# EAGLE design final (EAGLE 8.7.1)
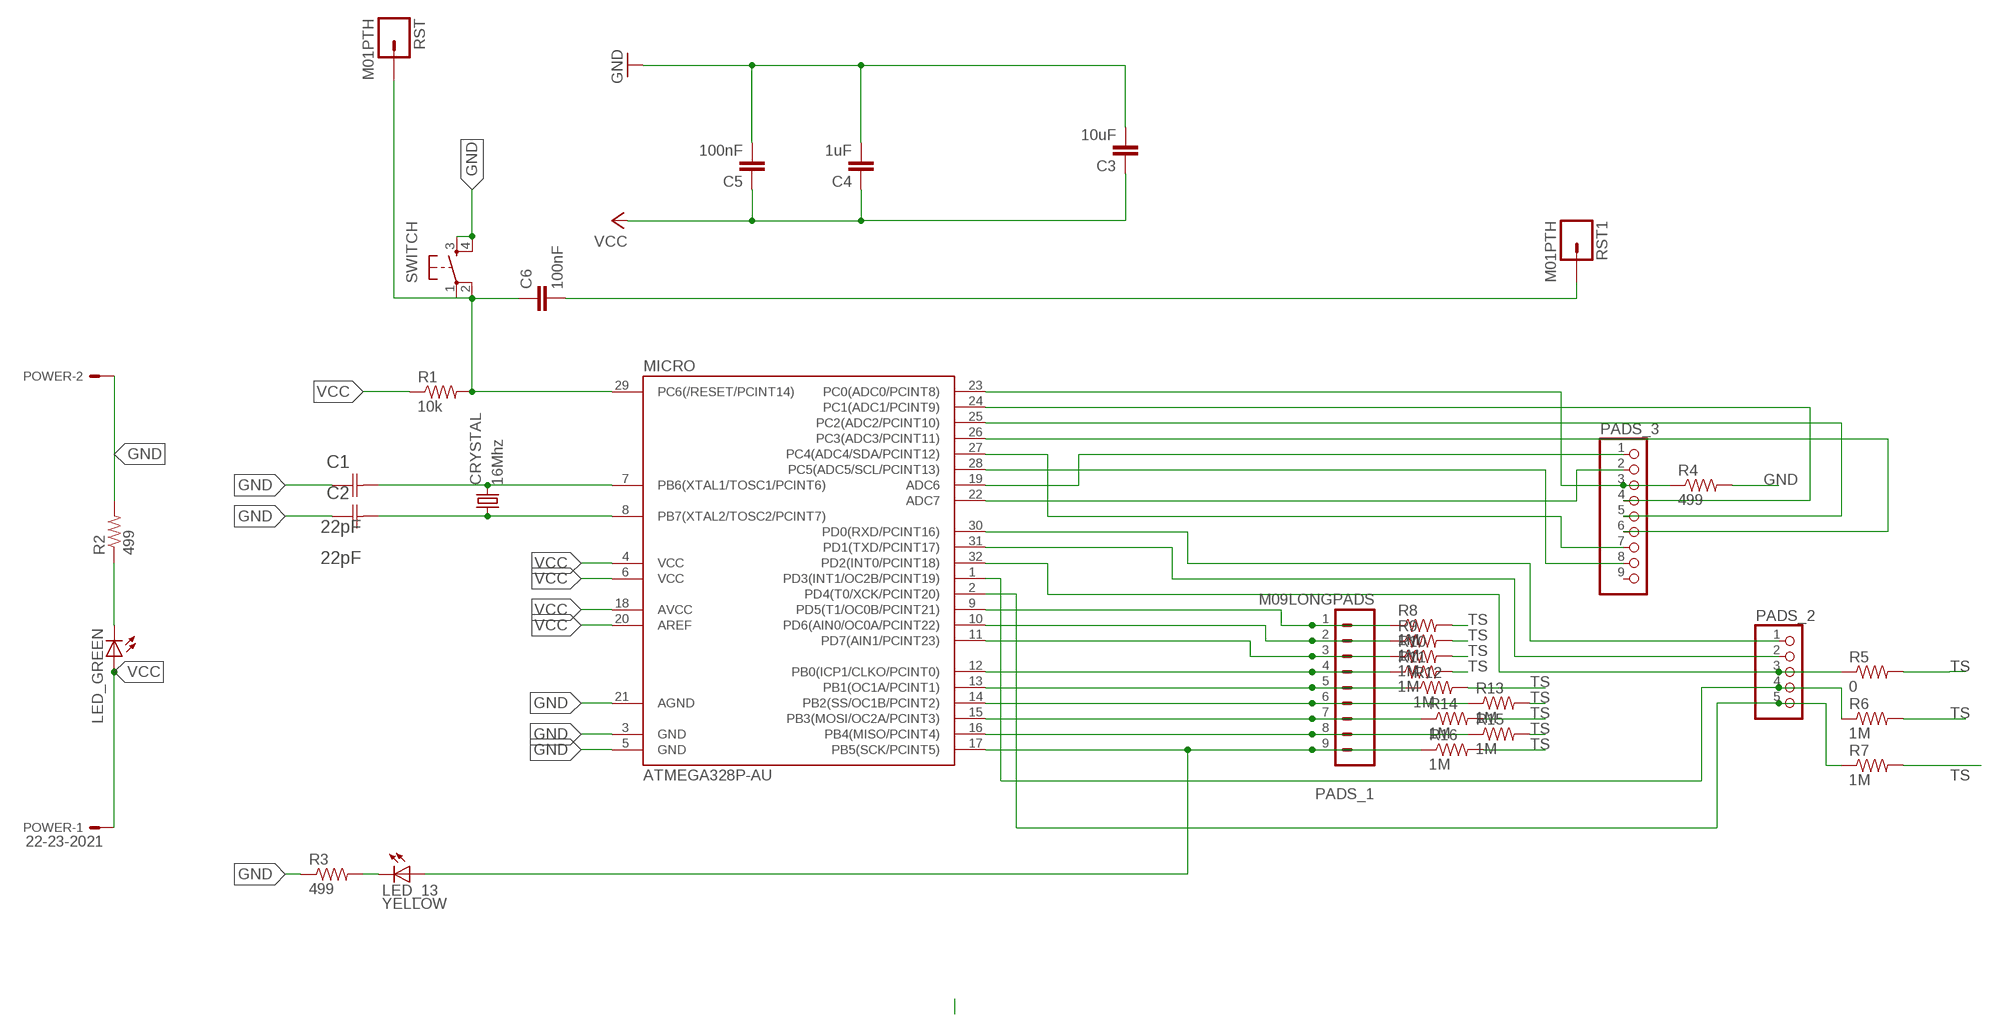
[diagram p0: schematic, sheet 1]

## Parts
C1  22pF  0612ZC225MAT2A  [CAPC3216X178N]
C2  22pF  0612ZC225MAT2A  [CAPC3216X178N]
C3  10uF  CAP1206  [1206]
C4  1uF  CAP1206  [1206]
C5  100nF  CAP1206  [1206]
C6  100nF  CAP1206  [1206]
CRYSTAL  16Mhz  CSM-7X-DU  [CSM-7X-DU]
LED_13  YELLOW  LED1206  [1206]
LED_GREEN  LED1206  [1206]
MICRO  ATMEGA328P-AU  ATMEGA48/88/168-AU  [TQFP32-08]
PADS_1  M09LONGPADS  [1X09_LONGPADS]
PADS_2  PINHD-1X5  [1X05]
PADS_3  PINHD-1X9  [1X09]
POWER  22-23-2021  [22-23-2021]
R1  10k  RESISTOR1206  [1206]
R2  499  RESISTOR1206  [1206]
R3  499  RESISTOR1206  [1206]
R4  499  RES-US1206FAB  [R1206FAB]
R5  0  RES-US1206FAB  [R1206FAB]
R6  1M  RES-US1206FAB  [R1206FAB]
R7  1M  RES-US1206FAB  [R1206FAB]
R8  1M  RES-US1206FAB  [R1206FAB]
R9  1M  RES-US1206FAB  [R1206FAB]
R10  1M  RES-US1206FAB  [R1206FAB]
R11  1M  RES-US1206FAB  [R1206FAB]
R12  1M  RES-US1206FAB  [R1206FAB]
R13  1M  RES-US1206FAB  [R1206FAB]
R14  1M  RES-US1206FAB  [R1206FAB]
R15  1M  RES-US1206FAB  [R1206FAB]
R16  1M  RES-US1206FAB  [R1206FAB]
RST  M01PTH  [1X01]
RST1  M01PTH  [1X01]
SWITCH  6MM_SWITCH6MM_SWITCH  [6MM_SWITCH]

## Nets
GND: C1.1(C1) C2.1(C1) C3.2 C4.2 C5.2 MICRO.3(GND) MICRO.5(GND) MICRO.21(AGND) POWER.2 R2.2 R3.1 R4.2 SWITCH.3(S) SWITCH.4(S1)
N$1: MICRO.9(PD5(T1/OC0B/PCINT21)) PADS_1.1 R8.1
N$2: C1.2(C2) CRYSTAL.2 MICRO.7(PB6(XTAL1/TOSC1/PCINT6))
N$4: MICRO.10(PD6(AIN0/OC0A/PCINT22)) PADS_1.2 R9.1
N$5: MICRO.11(PD7(AIN1/PCINT23)) PADS_1.3 R10.1
N$6: MICRO.12(PB0(ICP1/CLKO/PCINT0)) PADS_1.4 R11.1
N$7: MICRO.16(PB4(MISO/PCINT4)) PADS_1.8 R15.1
N$8: MICRO.15(PB3(MOSI/OC2A/PCINT3)) PADS_1.7 R14.1
N$9: C2.2(C2) CRYSTAL.1 MICRO.8(PB7(XTAL2/TOSC2/PCINT7))
N$10: MICRO.14(PB2(SS/OC1B/PCINT2)) PADS_1.6 R13.1
N$11: MICRO.13(PB1(OC1A/PCINT1)) PADS_1.5 R12.1
N$12: LED_13.1(A) MICRO.17(PB5(SCK/PCINT5)) PADS_1.9 R16.1
N$13: MICRO.19(ADC6) PADS_3.1
N$14: MICRO.22(ADC7) PADS_3.2
N$15: C6.2 RST1.1
N$16: MICRO.24(PC1(ADC1/PCINT9)) PADS_3.4
N$17: MICRO.25(PC2(ADC2/PCINT10)) PADS_3.5
N$18: MICRO.26(PC3(ADC3/PCINT11)) PADS_3.6
N$19: MICRO.27(PC4(ADC4/SDA/PCINT12)) PADS_3.7
N$20: MICRO.30(PD0(RXD/PCINT16)) PADS_2.1
N$21: MICRO.31(PD1(TXD/PCINT17)) PADS_2.2
N$25: MICRO.28(PC5(ADC5/SCL/PCINT13)) PADS_3.8
N$26: LED_GREEN.2(C) R2.1
N$27: LED_13.2(C) R3.2
N$28: C6.1 MICRO.29(PC6(/RESET/PCINT14)) R1.2 RST.1 SWITCH.1(P) SWITCH.2(P1)
N$29: MICRO.23(PC0(ADC0/PCINT8)) PADS_3.3 R4.1
N$30: MICRO.32(PD2(INT0/PCINT18)) PADS_2.3 R5.1
N$31: MICRO.1(PD3(INT1/OC2B/PCINT19)) PADS_2.4 R6.1
N$32: MICRO.2(PD4(T0/XCK/PCINT20)) PADS_2.5 R7.1
TS: R5.2 R6.2 R7.2 R8.2 R9.2 R10.2 R11.2 R12.2 R13.2 R14.2 R15.2 R16.2
VCC: C3.1 C4.1 C5.1 LED_GREEN.1(A) MICRO.4(VCC) MICRO.6(VCC) MICRO.18(AVCC) MICRO.20(AREF) POWER.1 R1.1
Unconnected: PADS_3.9

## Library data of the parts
C1 C2 = AVX_By_element14_Batch_1:0612ZC225MAT2A: Capacitor 1206; MPN: 0612ZC225MAT2A; OC_FARNELL: -; OC_NEWARK: 12N3209; SUPPLIER: AVX; TOLERANCE: ±20%; VALUE: 2.2µF; VOLTAGERATING: 10V
C3-C6 = 01_SparkFun:CAP: Capacitor
CRYSTAL = 01_FAB_Hello:CSM-7X-DU: SMD CRYSTAL; OC_FARNELL: unknown; OC_NEWARK: unknown
LED_13 LED_GREEN = 01_FAB_Hello:LED
MICRO = atmega8:ATMEGA48/88/168
PADS_1 = 01_SparkFun:M09: Header 9 Standard 9-pin 0.1" header. Use with straight break away headers (SKU : PRT-00116), right angle break away headers (PRT-00553), swiss pins (PRT-00743), machine pins (PRT-00117), and female headers (PRT-00115).
PADS_2 = pinhead:PINHD-1X5: PIN HEADER
PADS_3 = pinhead:PINHD-1X9: PIN HEADER
POWER = con-molex:22-23-2021: .100" (2.54mm) Center Header - 2 Pin; MF: MOLEX; MPN: 22-23-2021; OC_FARNELL: 1462926; OC_NEWARK: 25C3832
R1-R3 = 01_SparkFun:RESISTOR: Resistor
R4-R16 = 00fab:RES-US: Resistor (US Symbol)
RST RST1 = 01_SparkFun:M01: Header 1
SWITCH = 01_FAB_Hello:6MM_SWITCH: OMRON SWITCH

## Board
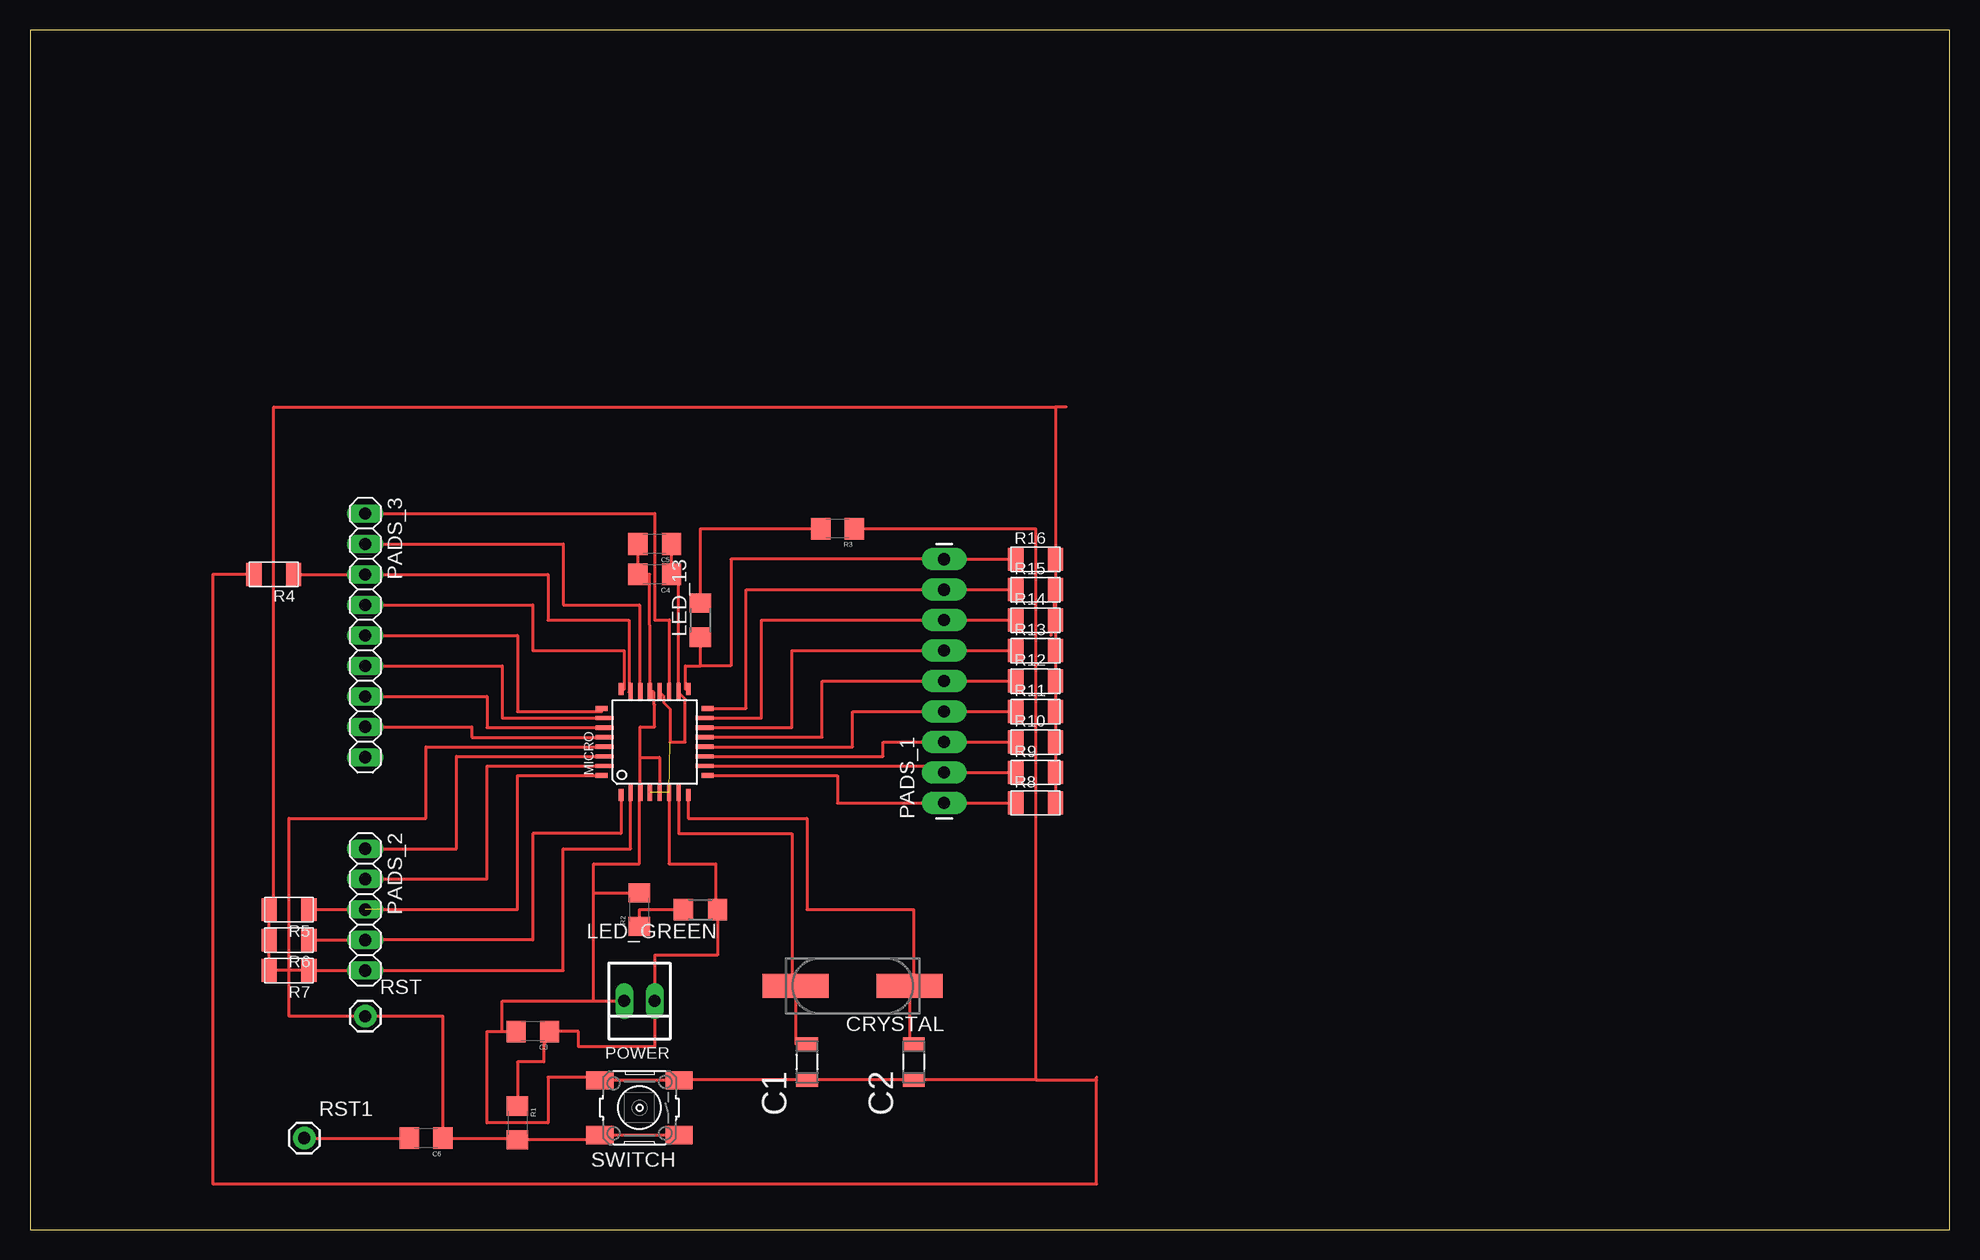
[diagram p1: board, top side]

Size 160 x 100 mm. Coordinates in mm from the lower left corner, seen from the top.
Outline: 0,0 160,0 160,100 0,100 0,0
Copper layers (1*16): Top 0.035mm / dielectric 1.5mm / Bottom 0.035mm
Design rules "default": minimum track width 6mil, minimum drill 0.35mm, track to track 6mil, track to pad 6mil, pad to pad 6mil, via to via 6mil, smd to smd 6mil, copper to edge 40mil, drill to drill 6mil, minimum pad ring 10mil, minimum via ring 8mil, stop-mask expansion 4mil, vias tented up to drill 0mil, thermal gap 10mil

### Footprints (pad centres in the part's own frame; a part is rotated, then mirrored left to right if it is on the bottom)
CAPC3216X178N = smd 1.118 x 1.803: 1 -1.499,0; 2 1.499,0
1206 = smd 1.6 x 1.8: 1 -1.4,0; 2 1.4,0
CSM-7X-DU = smd 5.5 x 2: 1 -4.75,0; 2 4.75,0
1206' = smd 1.6 x 1.803: 1 -1.422,0; 2 1.422,0
TQFP32-08 = smd 1.016 x 0.406: 1 -4.42,2.8; 8 -4.42,-2.8; 17 4.42,-2.8; 24 4.42,2.8 | smd 1.524 x 0.356: 2 -4.166,2; 3 -4.166,1.2; 4 -4.166,0.4; 5 -4.166,-0.4; 6 -4.166,-1.2; 7 -4.166,-2; 18 4.166,-2; 19 4.166,-1.2; 20 4.166,-0.4; 21 4.166,0.4; 22 4.166,1.2; 23 4.166,2 | smd 0.406 x 1.016: 9 -2.8,-4.42; 16 2.8,-4.42; 25 2.8,4.42; 32 -2.8,4.42 | smd 0.356 x 1.524: 10 -2,-4.166; 11 -1.2,-4.166; 12 -0.4,-4.166; 13 0.4,-4.166; 14 1.2,-4.166; 15 2,-4.166; 26 2,4.166; 27 1.2,4.166; 28 0.4,4.166; 29 -0.4,4.166; 30 -1.2,4.166; 31 -2,4.166
1X09_LONGPADS = drill 1.016 pad 1.88 long: 1 0,0; 2 2.54,0; 3 5.08,0; 4 7.62,0; 5 10.16,0; 6 12.7,0; 7 15.24,0; 8 17.78,0; 9 20.32,0
1X05 = drill 1.016 long: 1 -5.08,0; 2 -2.54,0; 3 0,0; 4 2.54,0; 5 5.08,0
1X09 = drill 1.016 long: 1 -10.16,0; 2 -7.62,0; 3 -5.08,0; 4 -2.54,0; 5 0,0; 6 2.54,0; 7 5.08,0; 8 7.62,0; 9 10.16,0
22-23-2021 = drill 1 long: 1 -1.27,0; 2 1.27,0
R1206FAB = smd 1.27 x 1.905: 1 -1.651,0; 2 1.651,0
1X01 = drill 1.016 pad 1.88: 1 0,0
6MM_SWITCH = smd 2.286 x 1.524: 1 -3.302,2.286; 2 3.302,2.286; 3 -3.302,-2.286; 4 3.302,-2.286

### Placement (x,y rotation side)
C1  64.77,13.97 90 top
C2  73.66,13.97 90 top
C3  41.91,16.51 180 top
C4  52.07,54.61 180 top
C5  52.07,57.15 180 top
C6  33.02,7.62 180 top
CRYSTAL  68.58,20.32 180 top
LED_13  YELLOW  [1206']  55.88,50.8 90 top
LED_GREEN  [1206']  55.88,26.67 180 top
MICRO  52.07,40.64 90 top
PADS_1  76.2,35.56 90 top
PADS_2  27.94,26.67 270 top
PADS_3  27.94,49.53 270 top
POWER  50.8,19.05 180 top
R1  40.64,8.89 270 top
R2  50.8,26.67 90 top
R3  67.31,58.42 180 top
R4  20.32,54.61 180 top
R5  21.59,26.67 180 top
R6  21.59,24.13 180 top
R7  21.59,21.59 180 top
R8  83.82,35.56 0 top
R9  83.82,38.1 0 top
R10  83.82,40.64 0 top
R11  83.82,43.18 0 top
R12  83.82,45.72 0 top
R13  83.82,48.26 0 top
R14  83.82,50.8 0 top
R15  83.82,53.34 0 top
R16  83.82,55.88 0 top
RST  27.94,17.78 0 top
RST1  22.86,7.62 0 top
SWITCH  50.8,10.16 180 top

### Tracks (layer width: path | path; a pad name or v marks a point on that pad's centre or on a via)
GND
  Top 0.254: R3.1 83.82,58.42 83.82,12.47 | 83.82,12.47 C2.1 C1.1 54.1,12.47 SWITCH.3 SWITCH.4 47.5,12.7 43.18,12.7 43.18,8.89 38.1,8.89 38.1,16.51 39.37,16.51 | 83.82,12.47 88.9,12.47 | 88.9,12.47 88.9,12.7 | 88.9,12.47 88.9,3.81 15.24,3.81 15.24,54.61 R4.2 | 50.87,39.37 MICRO.3 50.8,36.47 50.8,30.48 46.99,30.48 46.99,28.07 | MICRO.5 52.47,39.37 50.87,39.37 | 50.87,39.37 50.87,41.91 52.07,41.91 52.07,43.76 52.01,43.76 52.01,44.81 MICRO.21 51.67,50.39 51.66,50.39 51.66,54.61 C4.2 C5.2 | 39.37,16.51 C3.2 | 39.37,16.51 39.37,19.05 46.99,19.05 | 46.99,19.05 46.99,28.07 | 46.99,28.07 R2.2 | 46.99,19.05 POWER.2
N$1
  Top 0.254: MICRO.9 67.31,37.84 67.31,35.56 PADS_1.1 R8.1
N$2
  Top 0.254: MICRO.7 54.07,33.02 63.5,33.02 63.5,20.32 CRYSTAL.2 63.83,15.47 C1.2
N$4
  Top 0.254: MICRO.10 76.2,38.64 PADS_1.2 R9.1
N$5
  Top 0.254: MICRO.11 71.12,39.44 71.12,40.64 PADS_1.3 R10.1
N$6
  Top 0.254: MICRO.12 68.58,40.24 68.58,43.18 PADS_1.4 R11.1
N$7
  Top 0.254: MICRO.16 59.69,43.44 59.69,53.34 PADS_1.8 R15.1
N$8
  Top 0.254: MICRO.15 60.96,42.64 60.96,50.8 PADS_1.7 R14.1 82.55,50.8
N$9
  Top 0.254: MICRO.8 54.87,34.29 64.77,34.29 64.77,26.67 73.66,26.67 73.66,20.32 CRYSTAL.1 73.33,15.47 C2.2
N$10
  Top 0.254: MICRO.14 63.5,41.84 63.5,48.26 PADS_1.6 R13.1
N$11
  Top 0.254: MICRO.13 56.87,41.04 56.87,41.05 66.04,41.05 66.04,45.72 PADS_1.5 R12.1
N$12
  Top 0.254: 55.88,46.99 58.42,46.99 58.42,55.88 PADS_1.9 R16.1 | MICRO.17 54.61,45.06 54.61,46.99 55.88,46.99 | 55.88,46.99 LED_13.1
N$13
  Top 0.254: PADS_3.1 52.07,59.69 52.07,50.8 53.27,50.8 | 53.34,50.8 53.27,50.8 | 53.27,50.8 MICRO.19
N$14
  Top 0.254: PADS_3.2 44.45,57.15 44.45,52.07 50.8,52.07 50.8,44.81 MICRO.22
N$15
  Top 0.254: RST1.1 C6.2
N$16
  Top 0.254: PADS_3.4 41.91,52.07 41.91,48.26 49.53,48.26 49.53,45.06 MICRO.24
N$17
  Top 0.254: PADS_3.5 40.64,49.53 40.64,43.18 47.65,43.18 MICRO.25
N$18
  Top 0.254: PADS_3.6 39.37,46.99 39.37,42.64 MICRO.26
N$19
  Top 0.254: PADS_3.7 38.1,44.45 38.1,41.84 MICRO.27
N$20
  Top 0.254: PADS_2.1 35.56,31.75 35.56,39.44 MICRO.30
N$21
  Top 0.254: PADS_2.2 38.1,29.21 38.1,38.64 MICRO.31
N$25
  Top 0.254: PADS_3.8 36.83,41.91 36.83,41.04 MICRO.28
N$26
  Top 0.254: R2.1 50.8,26.67 LED_GREEN.2
N$27
  Top 0.254: LED_13.2 55.88,58.42 R3.2
N$28
  Top 0.254: SWITCH.1 SWITCH.2 47.5,7.49 R1.2 40.64,7.62 C6.1 34.42,17.78 RST.1 21.59,17.78 21.59,34.29 33.02,34.29 33.02,40.24 MICRO.29
N$29
  Top 0.254: R4.1 PADS_3.3 43.18,54.61 43.18,50.8 49.94,50.8 49.94,44.81 MICRO.23
N$30  (1 unrouted)
  Top 0.254: R5.1 29.21,26.67 | PADS_2.3 40.64,26.67 40.64,37.84 MICRO.32
N$31
  Top 0.254: R6.1 PADS_2.4 41.91,24.13 41.91,33.02 49.27,33.02 MICRO.1
N$32
  Top 0.254: 20.32,21.59 R7.1 PADS_2.5 44.45,21.59 44.45,31.75 50.07,31.75 MICRO.2
TS
  Top 0.254: R5.2 R6.2 R7.2 R5.2 | R15.2 R16.2 85.47,68.58 | R15.2 85.09,49.53 | R15.2 R14.2 R13.2 R12.2 R11.2 R10.2 R9.2 R8.2 | R5.2 20.32,26.67 20.32,68.58 85.47,68.58 | 86.36,68.58 85.47,68.58
VCC  (2 unrouted)
  Top 0.254: MICRO.20 52.81,44.46 52.81,43.93 53.34,43.4 53.34,40.64 54.61,40.64 54.61,44.21 54.07,44.75 MICRO.18 54.07,54.61 C4.1 C5.1 | 40.51,10.29 R1.1 40.64,13.97 42.81,13.97 42.81,15.4 C3.1 45.72,16.51 45.72,15.24 52.07,15.24 POWER.1 52.07,22.86 57.3,22.86 LED_GREEN.1 57.15,26.67 57.15,30.48 53.27,30.48 MICRO.6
